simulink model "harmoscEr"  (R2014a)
settings: Solver=ode45  StartTime=0.0  StopTime=20.0  RelTol=1e-3
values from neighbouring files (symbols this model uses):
  omega = 2*pi/(24*3600)    (= 7.27220521664e-05)    [foucault_call.m]    (also in GravWirk.m = 1)
undefined symbols (not defined in the file or in its folder): Daempf

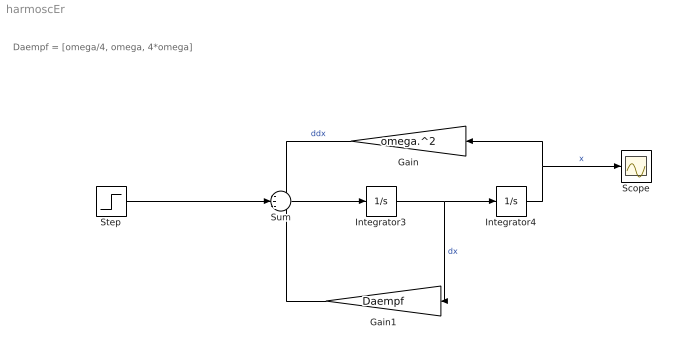
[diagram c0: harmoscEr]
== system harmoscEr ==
  note: Daempf = [omega/4, omega, 4*omega]
  Gain : Gain  Gain=omega.^2
  Gain1 : Gain  Gain=Daempf
  Integrator3 : Integrator
  Integrator4 : Integrator
  Scope : Scope
  Step : Step  SampleTime=0
  Sum : Sum  Inputs=-+-
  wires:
  Integrator3/1 -> Gain1/1, Integrator4/1  "dx"
  Integrator4/1 -> Scope/1, Gain/1  "x"
  Sum/1 -> Integrator3/1
  Gain/1 -> Sum/1  "ddx"
  Gain1/1 -> Sum/3
  Step/1 -> Sum/2
